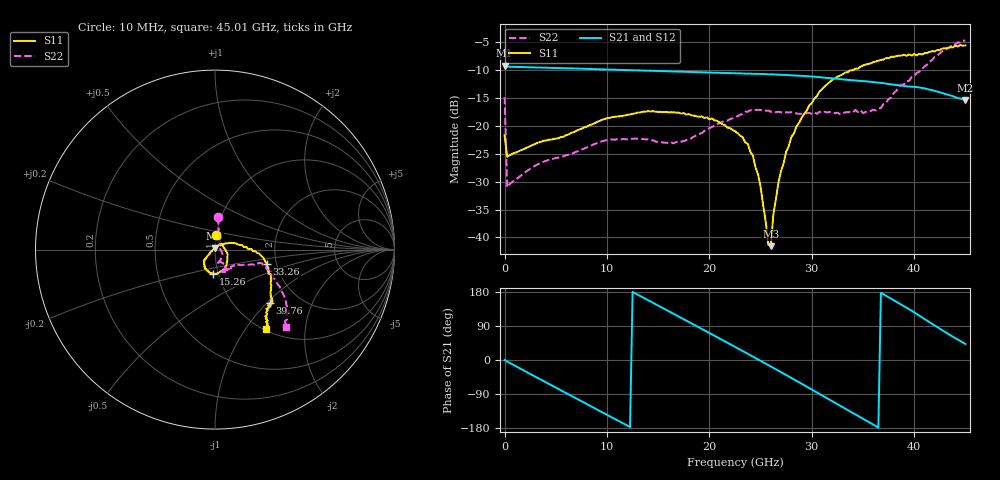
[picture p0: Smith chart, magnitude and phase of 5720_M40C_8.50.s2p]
! Device:  ADRF5720
! Description: 0.5dB LSB GaAs MMIC 6-bit Digital Attenuator
! Frequency:  0.000009 -  40 GHz
! Ports:
!	RF1	= Port 1
!	RF2	= Port 2
! Vdd:  3.3 Volt
! Vss:  -3.3 Volt
! Control:  0/3.3 Volt
! State:  8.50 dB attenuation
! Data:  The device was measured using G-S-G Probes on a matrix board.
!  Data was collected using an calibrated 4 port network analyzer.
!  The reference plane for this measurement is at the launchers.
! Note:  Analog Devices supplies this data as a sample of measured data
!  for this product.  Your particular data for this product may vary.
!  Data was taken at -40 degrees C.
!  Analog Devices reserves the right to change this data at anytime.
# GHZ S DB R 45.0
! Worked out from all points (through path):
!   181 points, 10 MHz to 45.01 GHz, reference 45 ohm
!   highest |S21| = -9.23 dB at 10 MHz (marker M1); lowest = -15.3 dB at 45.01 GHz (marker M2)
!   group delay of S21, straight-line fit = 41.5 ps
!   lowest |S11| = -41.6 dB at 26.01 GHz (marker M3), VSWR 1.02, Z = 44.8 + j0.725 ohm
!   |S11| at or under -10 dB: start of sweep to 34.05 GHz
!   |S22| runs from -31.0 to -4.7 dB; largest |S21 - S12| = 0.0013
!   S11 on the Smith chart (normalised r, x): 10 MHz: 0.99, +0.16; 15.26 GHz: 0.95, -0.26; 33.26 GHz: 1.78, -0.31; 39.76 GHz: 1.43, -1.04; 45.01 GHz: 1.03, -1.25
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0.01  -21.70 87.7  -9.23 -0.1  -9.25 -0.1  -14.87 84.9
0.26  -25.55 7.5  -9.40 -4.0  -9.41 -4.0  -31.03 13.8
4.26  -22.50 -20.1  -9.59 -62.1  -9.62 -62.1  -26.13 -33.5
7.76  -20.29 -45.7  -9.77 -112.4  -9.79 -112.4  -24.08 -59.6
11.51  -18.22 -70.0  -9.99 -166.2  -10.00 -166.2  -22.38 -77.0
15.26  -17.48 -94.4  -10.18 139.9  -10.20 139.9  -22.96 -80.0
19.01  -18.38 -114.5  -10.39 85.7  -10.41 85.7  -21.44 -60.6
22.76  -21.32 -135.6  -10.59 31.1  -10.62 31.0  -18.28 -63.3
24.26  -25.36 -139.0  -10.68 9.1  -10.70 9.0  -17.24 -66.6
25.01  -30.91 -152.4  -10.70 -2.1  -10.72 -2.2  -17.14 -67.2
25.76  -41.29 148.3  -10.76 -13.4  -10.78 -13.5  -17.26 -69.0
26.01  -41.56 104.6  -10.77 -17.1  -10.79 -17.2  -17.48 -70.0
26.26  -35.82 68.6  -10.78 -20.9  -10.81 -21.1  -17.43 -69.0
26.76  -30.03 51.7  -10.84 -28.4  -10.86 -28.6  -17.47 -69.8
27.51  -24.62 30.9  -10.88 -39.7  -10.91 -39.9  -17.56 -71.3
30.26  -15.10 4.9  -11.20 -81.9  -11.22 -82.0  -17.60 -67.6
33.26  -10.45 -15.4  -11.72 -127.9  -11.75 -128.0  -17.58 -56.8
36.26  -8.46 -34.5  -12.20 -174.6  -12.23 -174.7  -17.25 -38.2
37.76  -7.61 -40.7  -12.57 161.6  -12.59 161.4  -14.93 -28.1
39.76  -7.42 -44.5  -12.98 130.2  -13.00 130.0  -11.26 -16.1
42.26  -6.41 -52.8  -13.83 86.7  -13.85 86.5  -7.43 -31.0
45.01  -5.59 -57.1  -15.34 42.3  -15.37 42.1  -4.70 -47.5
